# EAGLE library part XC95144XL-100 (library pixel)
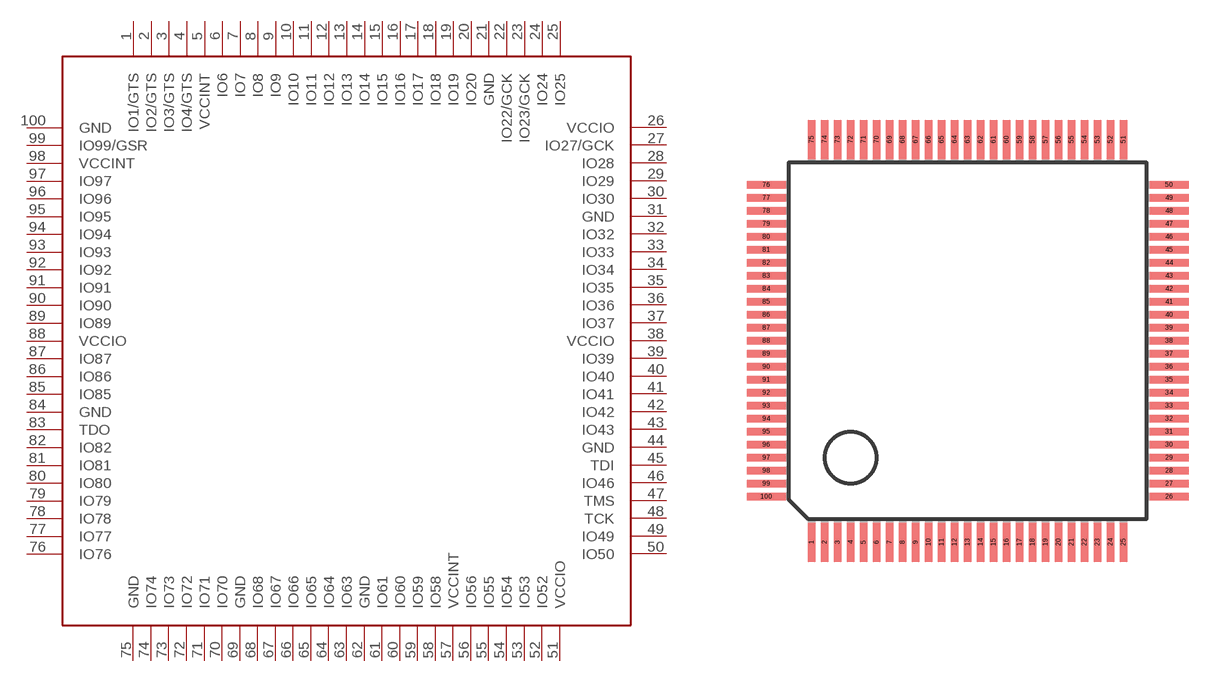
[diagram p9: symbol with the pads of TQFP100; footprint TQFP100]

Designator prefix -

## XC95144XL-100  [TQFP100]
1  IO1/GTS
2  IO2/GTS
3  IO3/GTS
4  IO4/GTS
5  VCCINT
6  IO6
7  IO7
8  IO8
9  IO9
10  IO10
11  IO11
12  IO12
13  IO13
14  IO14
15  IO15
16  IO16
17  IO17
18  IO18
19  IO19
20  IO20
21  GND
22  IO22/GCK
23  IO23/GCK
24  IO24
25  IO25
26  VCCIO
27  IO27/GCK
28  IO28
29  IO29
30  IO30
31  GND
32  IO32
33  IO33
34  IO34
35  IO35
36  IO36
37  IO37
38  VCCIO
39  IO39
40  IO40
41  IO41
42  IO42
43  IO43
44  GND
45  TDI
46  IO46
47  TMS
48  TCK
49  IO49
50  IO50
51  VCCIO
52  IO52
53  IO53
54  IO54
55  IO55
56  IO56
57  VCCINT
58  IO58
59  IO59
60  IO60
61  IO61
62  GND
63  IO63
64  IO64
65  IO65
66  IO66
67  IO67
68  IO68
69  GND
70  IO70
71  IO71
72  IO72
73  IO73
74  IO74
75  GND
76  IO76
77  IO77
78  IO78
79  IO79
80  IO80
81  IO81
82  IO82
83  TDO
84  GND
85  IO85
86  IO86
87  IO87
88  VCCIO
89  IO89
90  IO90
91  IO91
92  IO92
93  IO93
94  IO94
95  IO95
96  IO96
97  IO97
98  VCCINT
99  IO99/GSR
100  GND

## Footprint TQFP100 (pad centres in mm)
Thin Quad Flat Pack
smd 0.27 x 1.5: 1 -6,-7.75; 2 -5.5,-7.75; 3 -5,-7.75; 4 -4.5,-7.75; 5 -4,-7.75; 6 -3.5,-7.75; 7 -3,-7.75; 8 -2.5,-7.75; 9 -2,-7.75; 10 -1.5,-7.75; 11 -1,-7.75; 12 -0.5,-7.75; 13 0,-7.75; 14 0.5,-7.75; 15 1,-7.75; 16 1.5,-7.75; 17 2,-7.75; 18 2.5,-7.75; 19 3,-7.75; 20 3.5,-7.75; 21 4,-7.75; 22 4.5,-7.75; 23 5,-7.75; 24 5.5,-7.75; 25 6,-7.75; 51 6,7.75; 52 5.5,7.75; 53 5,7.75; 54 4.5,7.75; 55 4,7.75; 56 3.5,7.75; 57 3,7.75; 58 2.5,7.75; 59 2,7.75; 60 1.5,7.75; 61 1,7.75; 62 0.5,7.75; 63 0,7.75; 64 -0.5,7.75; 65 -1,7.75; 66 -1.5,7.75; 67 -2,7.75; 68 -2.5,7.75; 69 -3,7.75; 70 -3.5,7.75; 71 -4,7.75; 72 -4.5,7.75; 73 -5,7.75; 74 -5.5,7.75; 75 -6,7.75
smd 1.5 x 0.27: 26 7.75,-6; 27 7.75,-5.5; 28 7.75,-5; 29 7.75,-4.5; 30 7.75,-4; 31 7.75,-3.5; 32 7.75,-3; 33 7.75,-2.5; 34 7.75,-2; 35 7.75,-1.5; 36 7.75,-1; 37 7.75,-0.5; 38 7.75,0; 39 7.75,0.5; 40 7.75,1; 41 7.75,1.5; 42 7.75,2; 43 7.75,2.5; 44 7.75,3; 45 7.75,3.5; 46 7.75,4; 47 7.75,4.5; 48 7.75,5; 49 7.75,5.5; 50 7.75,6; 76 -7.75,6; 77 -7.75,5.5; 78 -7.75,5; 79 -7.75,4.5; 80 -7.75,4; 81 -7.75,3.5; 82 -7.75,3; 83 -7.75,2.5; 84 -7.75,2; 85 -7.75,1.5; 86 -7.75,1; 87 -7.75,0.5; 88 -7.75,0; 89 -7.75,-0.5; 90 -7.75,-1; 91 -7.75,-1.5; 92 -7.75,-2; 93 -7.75,-2.5; 94 -7.75,-3; 95 -7.75,-3.5; 96 -7.75,-4; 97 -7.75,-4.5; 98 -7.75,-5; 99 -7.75,-5.5; 100 -7.75,-6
